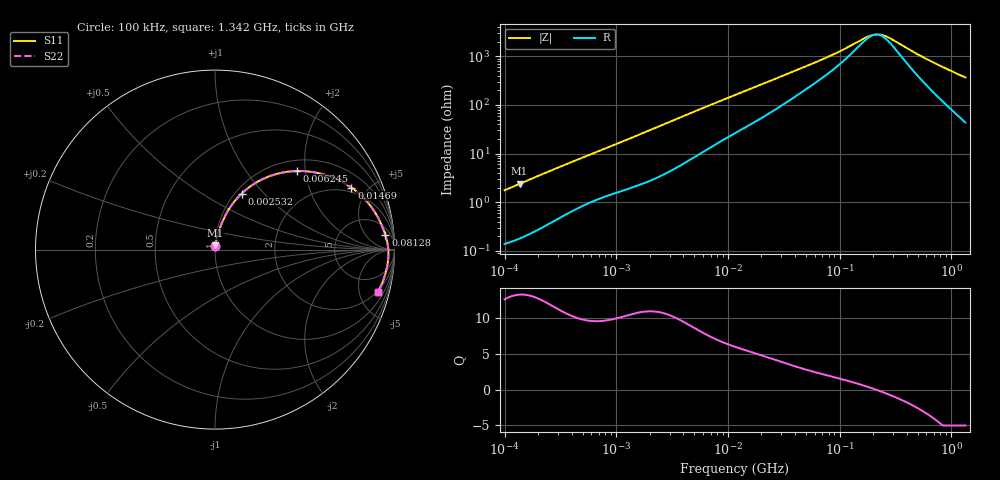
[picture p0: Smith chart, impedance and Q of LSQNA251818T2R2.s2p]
! LSQNA251818T2R2  S-PARAMETER MODEL  ( General Type )
! Model Generated by TAIYO YUDEN Corporation (http://www.ty-top.com)
! Version 2.0
! TAIYO YUDEN Control No. 100810NF25SB-FKC
! Copyright(c) 2007 TAIYO YUDEN CO.,LTD. All Rights Reserved.
! Product Description (link to TY-COMPAS)
! https://ds.yuden.co.jp/TYCOMPAS/or/detail?pn=LSQNA251818T2R2M&u=M
! Products Name : Inductors
! Characteristics :
!  Inductance : 2.2 uH , SRF(min) : 68 MHz , DC Resistance(max) : 0.117 Ohm
!  Rated Current : Saturation :510 mA , Temp Rise : 1300 mA (40 degC)
!  Case Size : 2.5 x 1.8 / 0.098 x 0.071 [mm/inch] , Thickness : 1.8 / 0.071 [mm/inch]
!  (Conditions: Temperature = 25 degC , DC Bias Current/Voltage = 0A / 0V)
! External Node Assignments :
!  1  o---GGG---o  2
! GND o---------o GND
! Frequency Range : 0.1MHz  -  1341.573064MHz  [ 402 STEP ]
# MHz S RI R 50
! Freq[MHz].  S11 Real  S11 Imag  S21 Real  S21 Imag  S12 Real  S12 Imag  S22 Real  S22 Imag
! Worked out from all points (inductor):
!   401 points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, 100 kHz to 1.342 GHz, reference 50 ohm
!   read as one part in series: L = 2.8 uH near 104.9 kHz
!   highest Q = 13.3 at 136.2 kHz (marker M1), where L = 2.8 uH
!   self-resonance near 212.1 MHz
!   S11 on the Smith chart (normalised r, x): 100 kHz: 1.00, +0.04; 2.532 MHz: 1.07, +0.76; 6.245 MHz: 1.23, +1.79; 14.69 MHz: 1.71, +3.91; 81.28 MHz: 10, +18; 1.342 GHz: 1.87, -7.28
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0.1  0.00171 0.0176  0.9983 -0.0176  0.9983 -0.0176  0.00171 0.0176
0.136191  0.00237 0.0238  0.9976 -0.0238  0.9976 -0.0238  0.00237 0.0238
0.491332  0.0146 0.0794  0.9854 -0.0794  0.9854 -0.0794  0.0146 0.0794
1.270974  0.0535 0.182  0.9465 -0.182  0.9465 -0.182  0.0535 0.182
2.414075  0.1383 0.3022  0.8617 -0.3022  0.8617 -0.3022  0.1383 0.3022
2.531564  0.1484 0.3121  0.8516 -0.3121  0.8516 -0.3121  0.1484 0.3121
3.791512  0.2613 0.3907  0.7387 -0.3907  0.7387 -0.3907  0.2613 0.3907
6.244709  0.4547 0.4379  0.5453 -0.4379  0.5453 -0.4379  0.4547 0.4379
8.30502  0.5704 0.4274  0.4296 -0.4274  0.4296 -0.4274  0.5704 0.4274
11.58263  0.6901 0.3865  0.3099 -0.3865  0.3099 -0.3865  0.6901 0.3865
14.68918  0.7602 0.3452  0.2398 -0.3452  0.2398 -0.3452  0.7602 0.3452
26.60562  0.8755 0.2314  0.1245 -0.2314  0.1245 -0.2314  0.8755 0.2314
56.90921  0.9359 0.1177  0.0641 -0.1177  0.0641 -0.1177  0.9359 0.1177
81.27708  0.9491 0.0802  0.0509 -0.0802  0.0509 -0.0802  0.9491 0.0802
165.7827  0.9634 0.0195  0.0366 -0.0195  0.0366 -0.0195  0.9634 0.0195
191.1848  0.9648 0.00824  0.0352 -0.00824  0.0352 -0.00824  0.9648 0.00824
210.2469  0.9655 0.000688  0.0345 -0.000688  0.0345 -0.000688  0.9655 0.000688
231.2095  0.9659 -0.00694  0.0341 0.00694  0.0341 0.00694  0.9659 -0.00694
279.6134  0.9662 -0.0226  0.0338 0.0226  0.0338 0.0226  0.9662 -0.0226
612.4719  0.9572 -0.1032  0.0428 0.1032  0.0428 0.1032  0.9572 -0.1032
961.9397  0.937 -0.172  0.063 0.172  0.063 0.172  0.937 -0.172
1341.573  0.9062 -0.2379  0.0938 0.2379  0.0938 0.2379  0.9062 -0.2379
